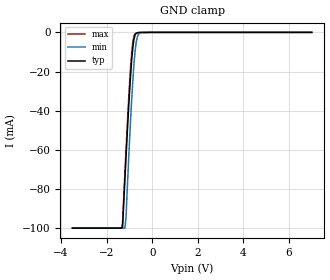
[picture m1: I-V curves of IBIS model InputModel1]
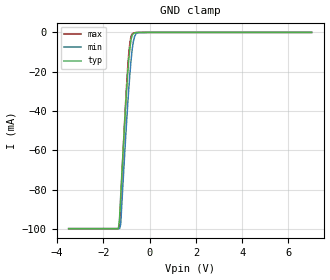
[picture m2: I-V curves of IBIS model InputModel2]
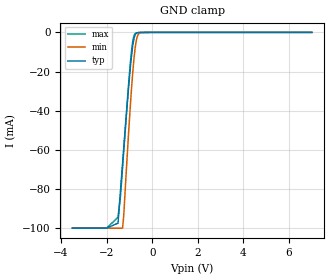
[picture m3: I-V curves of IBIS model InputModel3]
[IBIS Ver]   2.1
[File name]   pa200bv3.ibs   | pa= PSOP, f200bv= abbr chip name, 3= 3.3V Vcc
[File Rev]   2.00
[Date]   13-March-1996
[Source]   File generated from lab measurements at Intel Corporation
[Notes]   Rev 2.00 All data was replaced by actual measurements
   performed in a lab.
[Disclaimer] INTEL DEVELOPER'S SOFTWARE LICENSE AGREEMENT
| BY USING THIS SOFTWARE, YOU ARE AGREEING TO BE BOUND
| BY THE TERMS OF THIS AGREEMENT.  DO NOT USE THE SOFTWARE
| UNTIL YOU HAVE CAREFULLY READ AND AGREED TO THE FOLLOWING
| TERMS AND CONDITIONS.  IF YOU DO NOT AGREE TO THE TERMS
| OF THIS AGREEMENT, PROMPTLY RETURN THE SOFTWARE PACKAGE
| AND ANY ACCOMPANYING ITEMS.
| IF YOU USE THIS SOFTWARE, YOU WILL BE BOUND BY THE TERMS
| OF THIS AGREEMENT
| LICENSE: Intel Corporation ("Intel") grants you the non-exclusive right
| to use the enclosed software program ("Software").  You will not use,
| copy, modify, rent, sell or transfer the Software or any portion
| thereof, except as provided in this Agreement.
| System OEM Developers may:
| 1.   Copy the Software for support, backup or archival purposes;
| 2.   Install, use, or distribute Intel owned Software in object code
|   only;
| 3.   Modify and/or use Software source code that Intel directly makes
|   available to you as an OEM Developer;
| 4.   Install, use, modify, distribute, and/or make or have made
|   derivatives ("Derivatives") of Intel owned Software under the
|   terms and conditions in this Agreement, ONLY if you are a System
|   OEM Developer and NOT an end-user.
| RESTRICTIONS:
| YOU WILL NOT:
| 1.   Copy the Software, in whole or in part, except as provided for
|   in this Agreement;
| 2.   Decompile or reverse engineer any Software provided in object
|   code format;
| 3.   Distribute any Software or Derivative code to any end-users,
|   unless approved by Intel in a prior writing.
| TRANSFER: You may transfer the Software to another OEM
| Developer if the receiving party agrees to the terms of this
| Agreement at the sole risk of any receiving party.
| OWNERSHIP AND COPYRIGHT OF SOFTWARE:
| Title to the Software and all copies thereof remain with Intel
| or its vendors.  The Software is copyrighted and is protected by
| United States and international copyright laws.  You will not
| remove the copyright notice from the Software.  You agree to
| prevent any unauthorized copying of the Software.
| DERIVATIVE WORK: OEM Developers that make or have made
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[Copyright]   Copyright 1996, Intel Corporation, All Rights Reserved
[Component]   PA28F200BV   | 44-lead PSOP package, 28F200BV
[Manufacturer]  Intel   | Boot Block (tm)
|   | operating in 3.3V Vcc range
[Package]
R_pkg   145.5m   144.0m   147.0m
L_pkg   5.25nH   2.00nH   8.50nH
C_pkg   1.09pF   0.68pF   1.50pF
|*****************************Pin Definitions*****************************
[Pin]   signal_name   model_name   R_pin   L_pin   C_pin
 1   VPP   POWER
 2   WP#   InputModel1
 3   NC   InputModel3
 4   A07   InputModel3
 5   A06   InputModel3
 6   A05   InputModel3
 7   A04   InputModel3
 8   A03   InputModel3
 9   A02   InputModel1
10   A01   InputModel1
11   A00   InputModel2
12   CE#   InputModel1
13   GND   GND
14   OE#   InputModel1
15   DQ0   InputOutput
16   DQ8   InputOutput
17   DQ1   InputOutput
18   DQ9   InputOutput
19   DQ2   InputOutput
20   DQ10   InputOutput
21   DQ3   InputOutput
22   DQ11   InputOutput
23   VCC   POWER
24   DQ4   InputOutput
25   DQ12   InputOutput
26   DQ5   InputOutput
27   DQ13   InputOutput
28   DQ6   InputOutput
29   DQ14   InputOutput
30   DQ7   InputOutput
31   DQ15   InputOutput
32   GND   GND
33   BYTE#   InputModel2
34   A16   InputModel2
35   A15   InputModel3
36   A14   InputModel3
37   A13   InputModel3
38   A12   InputModel3
39   A11   InputModel3
40   A10   InputModel3
41   A09   InputModel3
42   A08   InputModel3
43   WE#   InputModel1
44   RP#   InputModel1
|***********************Input Model 4******************************
[Model]   InputModel4
Model_type   Input
|   Model for all NC pins, excluding NC pin #3.
Vinl = 0.8V
Vinh = 2.0V
|Variable   Typ   Min   Max
C_comp   4.91p   NA   6.50p
[Voltage Range]   3.3V   3.0V   3.6V
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| Models and submodels in the file (5): InputModel1 (Input), InputModel2 (Input), InputModel3 (Input), InputModel4 (Input), InputOutput (I/O)
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|*********************Input Model 1************************************
[Model]   InputModel1
Model_type   Input
|   Model for WE#, WP#, RP#, OE# & CE#.
Vinl = 0.8V
Vinh = 2.0V
|Variable   Typ   Min   Max
C_comp   4.91p   NA   6.50p
[Voltage Range]   3.3V   3.0V   3.6V
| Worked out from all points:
|   GND clamp passes 1 mA (typ) near -0.73 V on its own axis
[GND_clamp]
|Voltage  I(typ)   I(min)   I(max)
-3.5V     -99.85mA   -99.85mA   -99.85mA
-1.35V    -99.85mA   -99.85mA   -99.85mA
-1.3V     -99.26mA   -99.85mA   -97.14mA
-1.2V     -75.18mA   -99.85mA   -72.14mA
-1.15V    -63.89mA   -94.76mA   -60.07mA
-1V       -31.6mA    -56.54mA   -27.07mA
-900mV    -14.05mA   -34.26mA   -10.17mA
-850mV    -7.687mA   -24.68mA   -4.745mA
-750mV    -1.284mA   -9.549mA   -630.3uA
-650mV    -225.8uA   -2.279mA   -169.1uA
-500mV    -29.1uA    -152uA     -20.31uA
7V        0A         0A         0A
[Power_clamp]
| Input buffer circuits of this product do not intrinsically
| require a [Power_clamp] definition.  This zero current
| [Power_clamp] table is provided for the compatibility with
| some IBIS parsers.
|Voltage  I(typ)   I(min)   I(max)
-3.3V     0A         0A         0A
0V        0A         0A         0A
3.3V      0A         0A         0A
7V        0A         0A         0A
|*********************Input Model 2******************************
[Model]   InputModel2
Model_type   Input
|   Model for A[0], A[16] & BYTE# pins.
Vinl = 0.8V
Vinh = 2.0V
|Variable   Typ   Min   Max
C_comp   4.91p   NA   6.50p
[Voltage Range]   3.3V   3.0V   3.6V
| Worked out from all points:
|   GND clamp passes 1 mA (typ) near -0.73 V on its own axis
[GND_clamp]
|Voltage  I(typ)   I(min)   I(max)
-3.5V     -99.85mA   -99.83mA   -99.85mA
-1.35V    -99.85mA   -99.83mA   -99.85mA
-1.3V     -94.37mA   -99.83mA   -98.64mA
-1.25V    -82.89mA   -97.51mA   -85.83mA
-1.1V     -50.15mA   -66.04mA   -49.42mA
-950mV    -21.04mA   -36.93mA   -18.24mA
-900mV    -13.36mA   -28.31mA   -10.32mA
-850mV    -7.565mA   -20.57mA   -4.846mA
-750mV    -1.296mA   -8.199mA   -639.8uA
-650mV    -228.2uA   -2.043mA   -174.9uA
-500mV    -30.35uA   -138.9uA   -20.97uA
7V        0A         0A         0A
[Power_clamp]
| Input buffer circuits of this product do not intrinsically
| require a [Power_clamp] definition.  This zero current
| [Power_clamp] table is provided for the compatibility with
| some IBIS parsers.
|Voltage  I(typ)   I(min)   I(max)
-3.3V     0A         0A         0A
0V        0A         0A         0A
3.3V      0A         0A         0A
7V        0A         0A         0A
|***********************Input Model 3******************************
[Model]   InputModel3
Model_type   Input
|   Model for A[15:1] & NC pin #3.
Vinl = 0.8V
Vinh = 2.0V
|Variable   Typ   Min   Max
C_comp   4.91p   NA   6.50p
[Voltage Range]   3.3V   3.0V   3.6V
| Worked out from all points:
|   GND clamp passes 1 mA (typ) near -0.73 V on its own axis
[GND_clamp]
|Voltage  I(typ)   I(min)   I(max)
-3.5V     -99.85mA   -99.85mA   -99.84mA
-2V       -99.85mA   -99.85mA   -99.84mA
-1.5V     -97.31mA   -99.85mA   -94.31mA
-1.4V     -82.07mA   -99.85mA   -84.51mA
-1.3V     -66.84mA   -99.85mA   -68.9mA
-1.25V    -59.17mA   -93.69mA   -60.87mA
-950mV    -16.82mA   -35.79mA   -14.52mA
-850mV    -6.51mA    -20.05mA   -4.331mA
-750mV    -1.251mA   -8.08mA    -628.9uA
-650mV    -222.2uA   -2.03mA    -171.1uA
-500mV    -30.37uA   -137.4uA   -20.58uA
7V        0A         0A         0A
[Power_clamp]
| Input buffer circuits of this product do not intrinsically
| require a [Power_clamp] definition.  This zero current
| [Power_clamp] table is provided for the compatibility with
| some IBIS parsers.
|Voltage  I(typ)   I(min)   I(max)
-3.3V     0A         0A         0A
0V        0A         0A         0A
3.3V      0A         0A         0A
7V        0A         0A         0A
